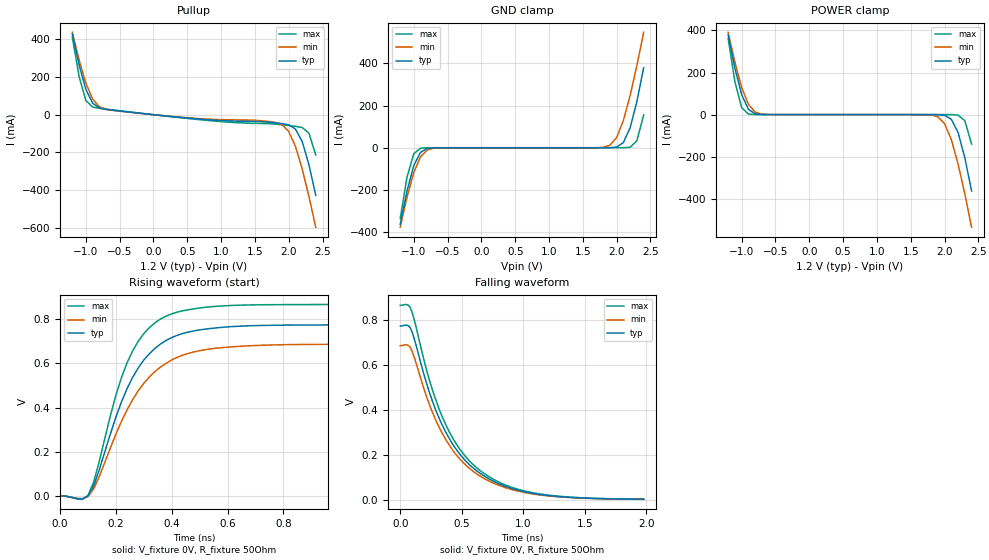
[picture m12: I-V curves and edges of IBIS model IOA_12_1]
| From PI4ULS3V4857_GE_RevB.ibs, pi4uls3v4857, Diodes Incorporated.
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[Model]  IOA_12_1
Model_type  Open_source
Vmeas=0.4
Vref=0
Rref=50
|Variable   typ   min   max
C_comp   4.38p   4.35p   4.41p
|Variable   typ   min   max
[Voltage Range]   1.2   1.1   1.3
[Temperature Range]   40   85   -40
[Pullup Reference]   1.2   1.1   1.3
[Power Clamp Reference]   1.2   1.1   1.3
[GND Clamp Reference]   0   0   0
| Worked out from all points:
|   slope of the pullup table from 0 to 0.18 V, typ, clamps not added: 26.7 ohm
|   GND clamp passes 1 mA (typ) near -0.72 V on its own axis
|   POWER clamp passes 1 mA (typ) near -0.72 V on its own axis
|   falling waveform, V_fixture 0V, R_fixture 50Ohm: 20-80 % time 401ps typ, 404ps min, 398ps max; typ from 0.773 V to 0.003 V
|   rising waveform, V_fixture 0V, R_fixture 50Ohm: 20-80 % time 154ps typ, 173ps min, 133ps max; typ from 0.002 V to 0.773 V
[GND Clamp]
-1.2V     -363mA     -377mA     -335mA
-1.1V     -205mA     -235mA     -140mA
-1V       -84.8mA    -118mA     -28.6mA
-900mV    -21.7mA    -42.8mA    -2.29mA
-800mV    -3.31mA    -10.4mA    -51.5uA
1.7V      183nA      121uA      6.42pA
1.9V      214uA      11.7mA     2.28nA
2V        3.47mA     48.5mA     315nA
2.1V      24.8mA     129mA      39.3uA
2.2V      94.6mA     248mA      2.33mA
2.3V      220mA      391mA      33mA
2.4V      380mA      548mA      156mA
[POWER Clamp]
-1.2V     380mA      391mA      362mA
-1.1V     220mA      248mA      156mA
-1V       94.7mA     129mA      33.1mA
-900mV    24.9mA     48.6mA     2.36mA
-800mV    3.5mA      11.7mA     65.4uA
-600mV    27uA       142uA      19.6uA
1.9V      -320uA     -10.4mA    -62.1uA
2V        -3.38mA    -42.8mA    -65.8uA
2.1V      -21.8mA    -118mA     -120uA
2.2V      -84.9mA    -235mA     -2.36mA
2.3V      -205mA     -377mA     -28.7mA
2.4V      -363mA     -535mA     -140mA
[Pullup]   |Note: Vtable = Vcc - Voutput
| Voltage   I(typ)   I(min)  I(max)
-1.2V     430mA      438mA      413mA
-1.1V     265mA      291mA      203mA
-1V       135mA      168mA      75.7mA
-900mV    61.3mA     83.3mA     40.7mA
-800mV    35.7mA     42.4mA     34mA
0V        3.48nA     37.2nA     15.4pA
1.9V      -47mA      -53.2mA    -53.7mA
2V        -53.9mA    -89.4mA    -57.6mA
2.1V      -76.2mA    -169mA     -61.8mA
2.2V      -143mA     -289mA     -68.2mA
2.3V      -267mA     -436mA     -98.8mA
2.4V      -429mA     -598mA     -214mA
[Falling Waveform]
V_fixture = 0V
V_fixture_min = 0V
V_fixture_max = 0V
R_fixture = 50Ohm
C_fixture = 0F
|   Time   V(typ)   V(min)   V(max)
0s        772.9mV    685.8mV    864.8mV
80ps      766.7mV    679.4mV    857mV
120ps     705.7mV    624.6mV    788.7mV
240ps     473.6mV    420.4mV    528mV
380ps     291.9mV    259.7mV    323.6mV
480ps     207.2mV    185.1mV    229.4mV
640ps     122.2mV    109.4mV    134.9mV
860ps     59.92mV    54.2mV     65.93mV
1.12ns    25.92mV    23.66mV    28.24mV
1.98ns    3.309mV    3.057mV    3.523mV
[Rising Waveform]
V_fixture = 0V
V_fixture_min = 0V
V_fixture_max = 0V
R_fixture = 50Ohm
C_fixture = 0F
|   Time   V(typ)   V(min)   V(max)
0s        2.002mV    1.845mV    2.119mV
100ps     1.778mV    -1.549mV   4.042mV
120ps     46.97mV    32.81mV    63.23mV
200ps     357.1mV    280.6mV    456mV
240ps     485.6mV    389.9mV    601.9mV
300ps     614.5mV    509.4mV    733.3mV
400ps     715.7mV    614.8mV    822.5mV
520ps     753.7mV    660.9mV    852.1mV
720ps     770.2mV    680.8mV    863.5mV
1.98ns    772.9mV    685.8mV    864.8mV
[Ramp]
|   typ   min   max
dV/dt_r   0.63/1.03E-10   0.56/1.16E-10   0.70/0.89E-10
dV/dt_f   0.62/4.03E-10   0.55/4.06E-10   0.69/4.00E-10
R_load =   50.0000
